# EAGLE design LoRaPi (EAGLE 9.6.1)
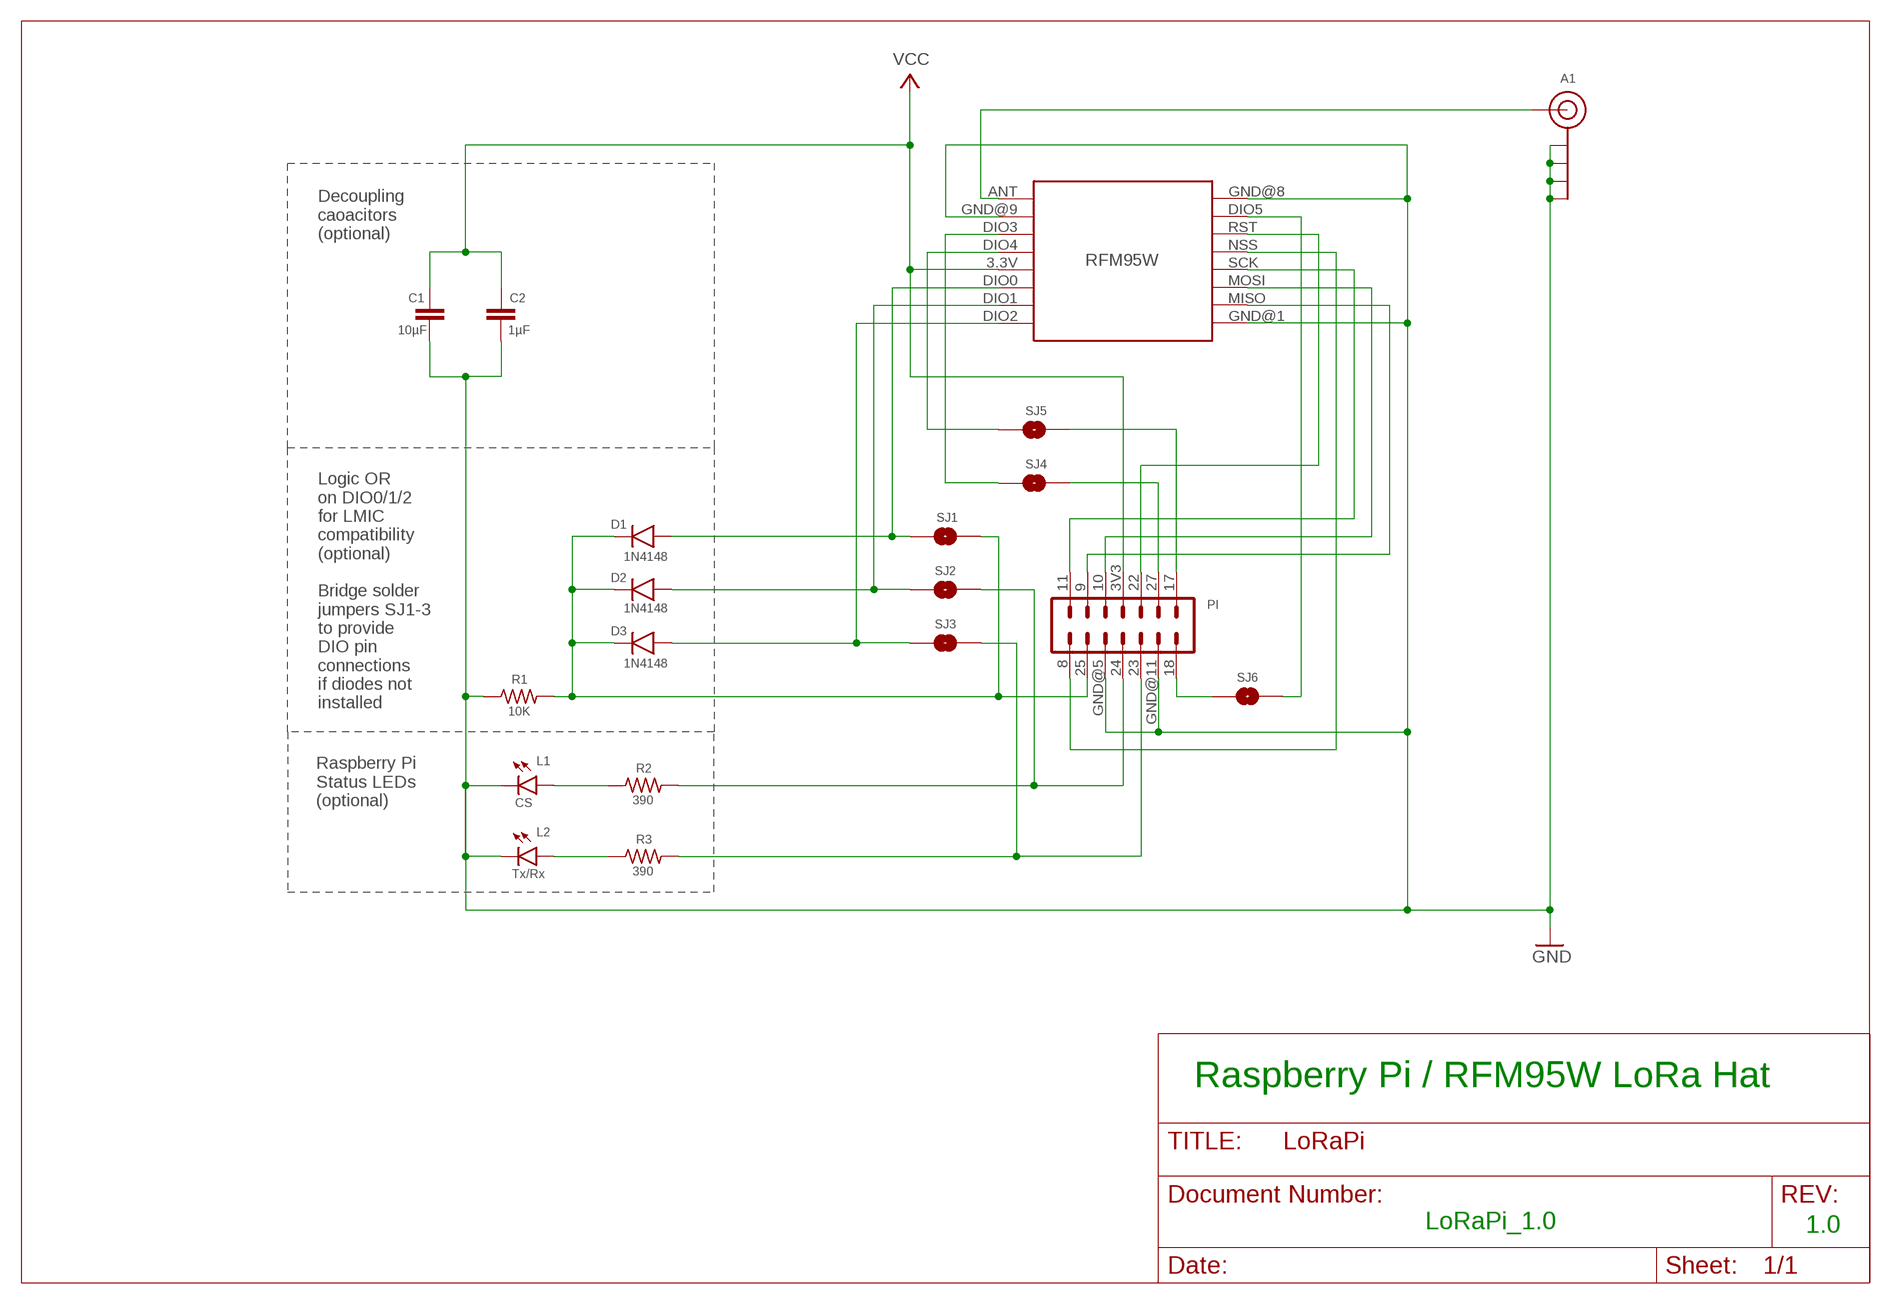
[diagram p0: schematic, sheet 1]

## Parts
A1  U.FL-SMA-EDGE-COMBO  [U.FL-SMA-EDGE-COMBO]
C1  10µF  CAPACITOR  [C0805]
C2  1µF  CAPACITOR  [C0805]
D1  1N4148  1N4148SMD  [SOD-123]
D2  1N4148  1N4148SMD  [SOD-123]
D3  1N4148  1N4148SMD  [SOD-123]
L1  CS  LEDCHIP-LED0805  [CHIP-LED0805]
L2  Tx/Rx  LEDCHIP-LED0805  [CHIP-LED0805]
PI  2X7-PIN-HEADER  [2X7]
R1  10K  R-US_R0805  [R0805]
R2  390  R-US_R0805  [R0805]
R3  390  R-US_R0805  [R0805]
RFM95W  RFM95W-LORA  [RFM95W-LORA]
SJ1  SJ  [SJ]
SJ2  SJ  [SJ]
SJ3  SJ  [SJ]
SJ4  SJ  [SJ]
SJ5  SJ  [SJ]
SJ6  SJ  [SJ]

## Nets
GND: A1.GND@1A(GND) A1.GND@1B(GND) A1.GND@2A(GND) A1.GND@2B(GND) C1.2 C2.2 L1.C L2.C PI.GND@5(GND) PI.GND@11(GND) R1.1 RFM95W.GND@1(GND.1) RFM95W.GND@8(GND.2) RFM95W.GND@9(GND.3)
N$1: L2.A R3.1
N$2: L1.A R2.1
N$3: PI.18 SJ6.1
N$4: PI.8 RFM95W.NSS
N$5: PI.23 R3.2 SJ3.2
N$6: PI.24 R2.2 SJ2.2
N$7: D1.2 RFM95W.DIO0 SJ1.1
N$8: RFM95W.DIO4 SJ5.1
N$9: RFM95W.DIO3 SJ4.1
N$10: D1.1 D2.1 D3.1 PI.25 R1.2 SJ1.2
N$11: A1.SIG RFM95W.ANT
N$12: D2.2 RFM95W.DIO1 SJ2.1
N$13: PI.22 RFM95W.RST
N$14: D3.2 RFM95W.DIO2 SJ3.1
N$15: PI.11 RFM95W.SCK
N$16: PI.10 RFM95W.MOSI
N$17: PI.9 RFM95W.MISO
N$18: PI.27 SJ4.2
N$19: PI.17 SJ5.2
N$20: RFM95W.DIO5 SJ6.2
VCC: C1.1 C2.1 PI.3V3 RFM95W.3.3V

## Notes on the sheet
- Decoupling
  caoacitors
  (optional)
- Logic OR
  on DIO0/1/2
  for LMIC
  compatibility
  (optional)
  
  Bridge solder
  jumpers SJ1-3
  to provide
  DIO pin
  connections
  if diodes not
  installed
- Raspberry Pi
  Status LEDs
  (optional)
- Raspberry Pi / RFM95W LoRa Hat
- LoRaPi_1.0 | 1.0

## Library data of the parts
A1 = digitalconcepts:U.FL-SMA-EDGE-COMBO: Combination u.FL & SMA edge mount antenna
C1 C2 = digitalconcepts:CAPACITOR: 0805 Capacitor
D1-D3 = digitalconcepts:1N4148: 1N4148 SOD-123 Signal Diode
L1 L2 = led:LED: LED
PI = digitalconcepts:2X7-PIN-HEADER: Double Row 14-Pin Header
R1-R3 = digitalconcepts:R-US_: RESISTOR, American symbol; SPICEPREFIX: R
RFM95W = digitalconcepts:RFM95W-LORA: RFM95W LoRa Wireless Transceiver
SJ1-SJ6 = digitalconcepts:SJ: Solder Jumper

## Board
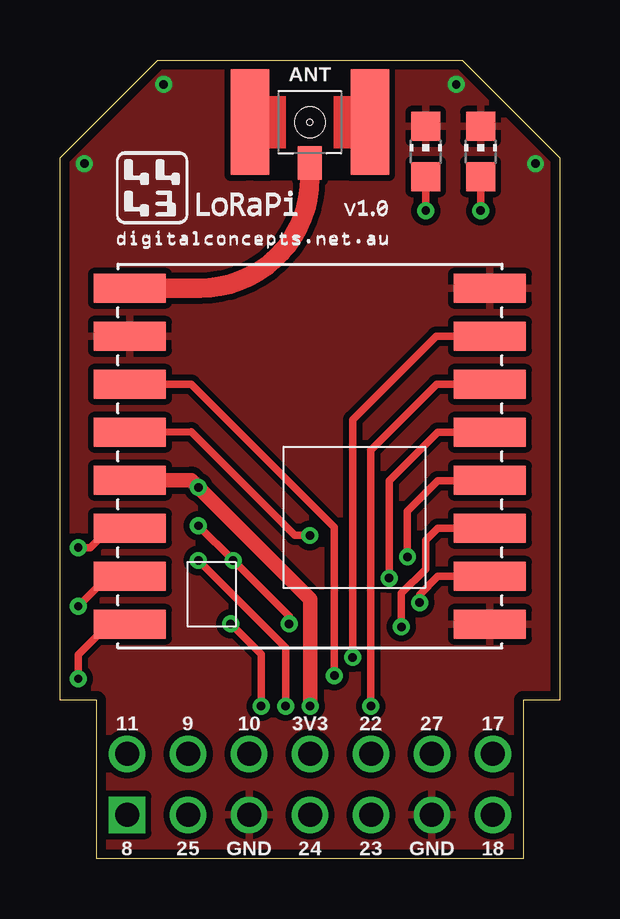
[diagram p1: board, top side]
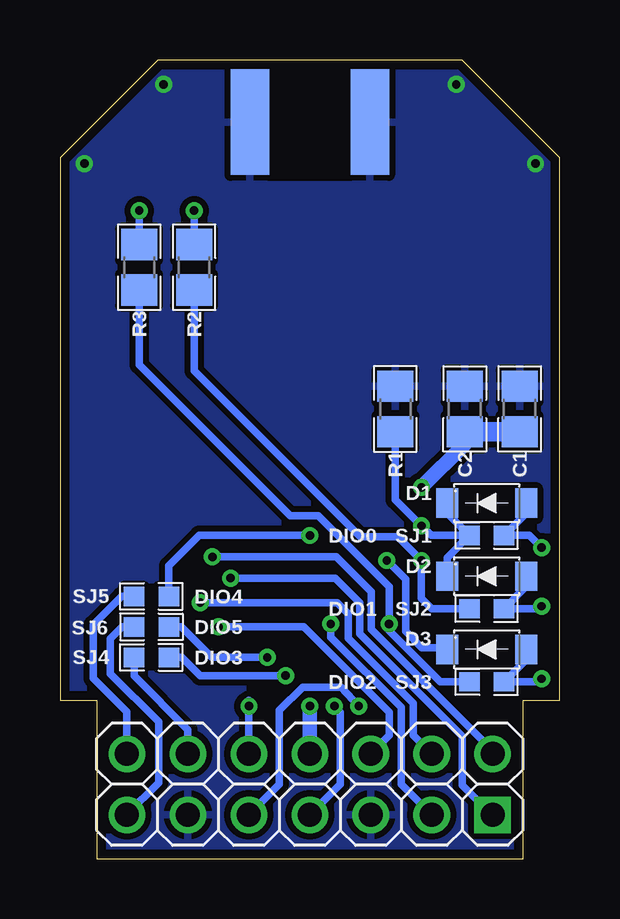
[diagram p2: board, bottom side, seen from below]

Size 20.83 x 33.27 mm. Coordinates in mm from the lower left corner, seen from the top.
Outline: 0,6.6 0,29.21 4.06,33.27 16.76,33.27 20.83,29.21 20.83,6.6 19.3,6.6 19.3,0 1.52,0 1.52,6.6 0,6.6
Copper layers (1*16): Top 0.0356mm / dielectric 1.5011mm / Bottom 0.0356mm
Design rules "PCBs_io": minimum track width 6mil, minimum drill 13mil, track to track 6mil, track to pad 6mil, pad to pad 6mil, via to via 6mil, smd to smd 6mil, copper to edge 15mil, drill to drill 6mil, minimum pad ring 7mil, minimum via ring 7mil, stop-mask expansion 3mil, vias tented up to drill 0mil, thermal gap 10mil

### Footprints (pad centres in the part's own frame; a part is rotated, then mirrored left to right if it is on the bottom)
U.FL-SMA-EDGE-COMBO = smd 1.6 x 4.4: GND@1A -2.5,0; GND@2A 2.5,0 | smd 1.6 x 4.4 bottom: GND@1B -2.5,0; GND@2B 2.5,0 | smd 1 x 1.4: SIG 0,-1.7
C0805 = smd 1.3 x 1.5: 1 -0.95,0; 2 0.95,0
SOD-123 = smd 0.91 x 1.22: 1 1.65,0; 2 -1.65,0
CHIP-LED0805 = smd 1.2 x 1.2: A 0,-1.05; C 0,1.05
2X7 = drill 1 pad 1.524: 3V3 7.62,2.54; 9 2.54,2.54; 10 5.08,2.54; 11 0,2.54; 17 15.24,2.54; 18 15.24,0; 22 10.16,2.54; 23 10.16,0; 24 7.62,0; 25 2.54,0; 27 12.7,2.54; GND@5 5.08,0; GND@11 12.7,0 | drill 1 pad 1.524 square: 8 0,0
R0805 = smd 1.3 x 1.5: 1 -0.95,0; 2 0.95,0
RFM95W-LORA = smd 3 x 1.2: 3.3V 7.5,1; ANT 7.5,-7; DIO0 7.5,3; DIO1 7.5,5; DIO2 7.5,7; DIO3 7.5,-3; DIO4 7.5,-1; DIO5 -7.5,-5; GND@1 -7.5,7; GND@8 -7.5,-7; GND@9 7.5,-5; MISO -7.5,5; MOSI -7.5,3; NSS -7.5,-1; RST -7.5,-3; SCK -7.5,1
SJ = smd 0.85 x 0.8: 1 -0.725,0; 2 0.725,0

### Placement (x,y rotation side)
A1  10.41,30.68 0 top
C1  1.68,18.74 90 bottom
C2  3.96,18.74 90 bottom
D1  3.05,14.81 180 bottom
D2  3.05,11.76 180 bottom
D3  3.05,8.71 180 bottom
L1  15.24,29.46 0 top
L2  17.53,29.46 0 top
PI  2.8,1.82 0 top
R1  6.86,18.74 270 bottom
R2  15.24,24.64 270 bottom
R3  17.53,24.64 270 bottom
RFM95W  10.41,16.76 180 top
SJ1  3.05,13.46 180 bottom
SJ2  3.05,10.41 180 bottom
SJ3  3.05,7.37 180 bottom
SJ4  17.02,8.38 180 bottom
SJ5  17.02,10.92 180 bottom
SJ6  17.02,9.65 0 bottom

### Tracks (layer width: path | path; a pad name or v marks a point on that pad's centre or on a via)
GND  (via drill 0.35)
  other vias: 1.02,28.96 4.32,32.26 16.51,32.26 19.81,28.96
  pour Top (isolate 0.254): 4.06,33.27 16.76,33.27 20.83,29.21 20.83,6.6 19.3,6.6 19.3,0 1.52,0 1.52,6.6 0,6.6 0,29.21
  pour Bottom (isolate 0.254): 4.06,33.27 16.76,33.27 20.83,29.21 20.83,6.6 19.3,6.6 19.3,0 1.52,0 1.52,6.6 0,6.6 0,29.21
N$1  (via drill 0.35)
  Top 0.305: L2.A v17.53,27
  Bottom 0.305: R3.1 v17.53,27
N$2  (via drill 0.35)
  Top 0.305: L1.A v15.24,27
  Bottom 0.305: R2.1 v15.24,27
N$3
  Bottom 0.305: PI.18 18.04,1.84 16.72,3.16 16.72,5.69 18.73,7.7 18.73,9.16 18.24,9.65 SJ6.1
N$4  (via drill 0.35)
  Top 0.305: v13.72,11.68 13.72,15.75 15.73,17.76 RFM95W.NSS
  Bottom 0.305: v13.72,11.68 9.36,11.68 8.34,10.67 8.34,9.37 4.06,5.09 4.06,3.05 2.84,1.82 PI.8
N$5  (via drill 0.35)
  Top 0.305: v7.11,9.78 8.38,8.51 v8.38,6.35
  Bottom 0.305: SJ3.2 4.99,7.37 7.11,9.49 v7.11,9.78 7.11,11.32 10.07,14.28 11.23,14.28 17.53,20.57 R3.2 | PI.23 11.68,3.1 11.68,6.17 10.72,7.13 9.12,7.13 v8.38,6.35
N$6  (via drill 0.35)
  Top 0.305: v5.77,12.42 9.4,8.79 v9.4,6.35
  Bottom 0.305: SJ2.2 5.33,10.41 5.77,10.85 v5.77,12.42 6.75,13.41 8.32,13.41 15.24,20.32 R2.2 | PI.24 9.14,3.1 9.14,6.1 v9.4,6.35
N$7  (via drill 0.35)
  Top 0.305: 2.03,13.76 2.03,13.72 1.27,12.95 v0.76,12.95
  Top 0.406: 2.03,13.76 RFM95W.DIO0
  Bottom 0.305: v0.76,12.95 1.27,13.46 SJ1.1 1.4,14.39 D1.2
N$8  (via drill 0.35)
  Top 0.305: RFM95W.DIO4 5.47,17.78 9.79,13.46 v10.41,13.46
  Bottom 0.305: v10.41,13.46 15.03,13.46 16.29,12.2 SJ5.1
N$9  (via drill 0.35)
  Top 0.305: v11.43,7.62 11.43,13.8 5.47,19.76 RFM95W.DIO3
  Bottom 0.305: SJ4.1 15.75,8.38 14.99,7.62 v11.43,7.62
N$10  (via drill 0.35)
  Top 0.305: v5.77,13.87 v7.21,12.42 9.55,10.09 v9.55,9.78
  Bottom 0.152: D3.1 4.76,8.78
  Bottom 0.305: v9.55,9.78 9.55,9.22 6.62,6.29 6.62,3.1 PI.25 | SJ1.2 4.7,12.54 D2.1 | D1.1 4.7,14.39 SJ1.2 | 4.76,8.78 5.75,8.78 6.43,9.46 6.43,11.64 v7.21,12.42 | R1.2 6.86,14.96 v5.77,13.87 5.36,13.46 SJ1.2
N$11
  Top 0.813: A1.SIG 10.41,28.48 10.4,28.34 arc-90 5.82,23.76 RFM95W.ANT
N$12  (via drill 0.35)
  Top 0.305: RFM95W.DIO1 1.78,11.76 1.78,11.53 v0.76,10.52
  Bottom 0.305: v0.76,10.52 0.86,10.41 SJ2.1 1.4,11.34 D2.2
N$13  (via drill 0.35)
  Top 0.305: v12.95,6.35 12.95,17.02 15.7,19.76 RFM95W.RST
  Bottom 0.305: v12.95,6.35 12.96,6.6 PI.22
N$14  (via drill 0.35)
  Top 0.152: RFM95W.DIO2 2.03,9.76
  Top 0.305: v0.76,7.49 0.76,8.49 2.03,9.76
  Bottom 0.305: v0.76,7.49 0.96,7.37 SJ3.1 1.4,8.29 D3.2
N$15  (via drill 0.35)
  Top 0.305: v14.48,12.57 14.48,14.48 15.75,15.75 17.9,15.75 RFM95W.SCK
  Bottom 0.305: PI.11 2.8,4.49 7.87,9.56 7.87,11.12 9.32,12.57 v14.48,12.57
N$16  (via drill 0.35)
  Top 0.305: RFM95W.MOSI 15.75,13.76 15.24,13.26 15.24,12.06 14.22,11.05 v14.22,9.65
  Bottom 0.305: PI.10 7.11,5.13 7.11,6.1 10.68,9.65 v14.22,9.65
N$17  (via drill 0.35)
  Top 0.305: RFM95W.MISO 15.75,11.76 14.99,11 v14.99,10.67
  Bottom 0.305: v14.99,10.67 9.28,10.67 8.81,10.21 8.81,9.18 6.11,6.47 6.11,5.13 PI.9
N$18
  Bottom 0.305: PI.27 15.5,5.38 17.74,7.62 SJ4.2
N$19
  Bottom 0.305: PI.17 18.04,6.11 19.44,7.51 19.44,9.73 18.25,10.92 SJ5.2
N$20  (via drill 0.35)
  Top 0.305: RFM95W.DIO5 15.67,21.76 12.19,18.29 v12.19,8.38
  Bottom 0.305: SJ6.2 15.78,9.65 14.52,8.38 v12.19,8.38
VCC  (via drill 0.35)
  Top 0.305: 10.42,10.81 10.42,10.8
  Top 0.61: 10.42,10.8 v10.42,6.35 | RFM95W.3.3V 5.47,15.76 v5.77,15.47 10.42,10.81
  Bottom 0.61: C2.1 3.96,17.27 v5.77,15.47 | PI.3V3 v10.42,6.35
  Bottom 0.813: C1.1 C2.1

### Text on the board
tPlace: ANT | 11 | 9 | 10 | 3V3 | 22 | 27 | 17 | 8 | 25 | GND | 24 | 23 | GND | 18
bPlace: DIO0 | DIO4 | DIO1 | DIO5 | DIO3 | DIO2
